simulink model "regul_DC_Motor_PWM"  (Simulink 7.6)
settings: Solver=ode15s  StartTime=0.0  StopTime=400  AbsTol=1e9
InitFcn:
  | clc, close all
  | N=400;
StopFcn:
  | load regul_vit_PWM.mat
  | 
  | plot(x(1,:),x(3,:), x(1,:),x(5,:))
  | grid
  | title('Consigne et sortie vitesse -  moteur DC  par pont en H et PWM')
  | xlabel('temps')
  | 
  | figure
  | plot(x(1,:),x(4,:))
  | grid
  | title('Signal de commande')
  | xlabel('temps')
  | 
  | figure
  | plot(x(1,:),x(2,:))
  | grid
  | axis([0 N -0.2 5.2])
  | title('Tension de commande PWM')
  | xlabel('temps')
undefined symbols (not defined in the file or in its folder): sigbuilder_block
libraries: fl_lib x19, nesl_utility x5, elec_lib x3

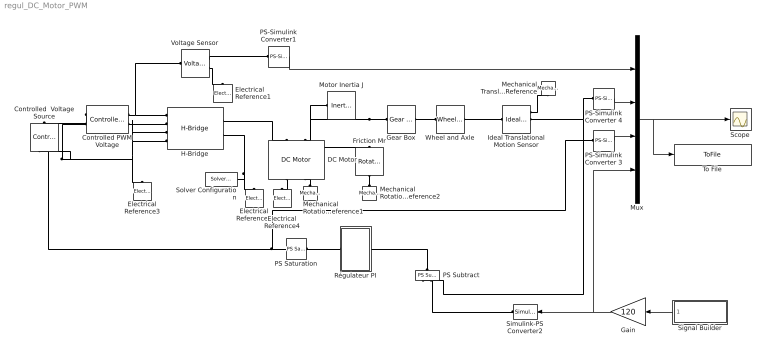
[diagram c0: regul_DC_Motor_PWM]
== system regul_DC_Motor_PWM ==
  Controlled  Voltage Source : fl_lib/Electrical/Electrical Sources/Controlled Voltage Source  DialogController=NetworkEngine.DynNeDlgSource  SystemSampleTime=-1  i_Log=off  v_Log=off  LocalVarNames=|i|v  LocalVarDescs=|i|v  LocalVarLogging=[0 0]
  Controlled PWM Voltage : elec_lib/Actuators & Drivers/Drivers/Controlled PWM Voltage  DialogController=NetworkEngine.DynNeDlgSource  SystemSampleTime=-1  F=200 Hz  Vmin=0 V  Vmax=5 V  Vm=5 V  pwm_or_av=1  current_Log=off  voltage_Log=off  power_Log=off  LocalVarNames=|current|voltage|power  LocalVarDescs=|Load current (A)|Load voltage (V)|Load power (W)  LocalVarLogging=[0 0 0]
  DC Motor : elec_lib/Actuators & Drivers/Rotational Actuators/DC Motor  DialogController=NetworkEngine.DynNeDlgSource  SystemSampleTime=-1  parameterization=1  Ra=3.9 Ohm  La=1.2e-05 H  emf_or_torque=1  Kv=7.2e-05 V/rpm  Ki=6.876e-04 N*m/A  T_stall=2.4e-04 N*m  w_max=1.91e+04 rpm  w_rated=1.5e+04 rpm  P_rated=0.08 W  V_rated=1.5 V  J=0.01 g*cm^2  lam=1e-08 N*m/(rad/s)  speed0=0 rpm  current_Log=off  voltage_Log=off  power_Log=off  i2r_Log=off  torque_Log=off  speed_Log=off  LocalVarNames=|current|voltage|power|i2r|torque|speed  LocalVarDescs=|Current (A)|Voltage (V)|Power (W)|Electrical losses (W)|Torque (Nm)|Angular speed (rad/s)  LocalVarLogging=[0 0 0 0 0 0]
  Electrical Reference{1..4} (4 alike) : fl_lib/Electrical/Electrical Elements/Electrical Reference  DialogController=NetworkEngine.DynNeDlgSource  SystemSampleTime=-1  i_Log=off  LocalVarNames=|i  LocalVarDescs=|i  LocalVarLogging=[]
  Friction Mr : fl_lib/Mechanical/Rotational Elements/Rotational Friction  DialogController=NetworkEngine.DynNeDlgSource  SystemSampleTime=-1  brkwy_trq=0.02e-3 N*m  Col_trq=0.02e-3 N*m  visc_coef=0 N*m/(rad/s)  trans_coef=10 s/rad  vel_thr=0.1 rad/s  t_Log=off  w_Log=off  LocalVarNames=|friction_torque|rel_velocity|power  LocalVarDescs=|Friction torque (N*m)|Relative velocity (rad/s)|Power (W)  LocalVarLogging=[0 0 0]
  Gain : Gain  Gain=120
  Gear Box : fl_lib/Mechanical/Mechanisms/Gear Box  DialogController=NetworkEngine.DynNeDlgSource  SystemSampleTime=-1  ratio=5  t_in_Log=off  t_out_Log=off  LocalVarNames=|t_in|t_out  LocalVarDescs=|t_in|t_out  LocalVarLogging=[0 0]
  H-Bridge : elec_lib/Actuators & Drivers/Drivers/H-Bridge  DialogController=NetworkEngine.DynNeDlgSource  SystemSampleTime=-1  Venable=2.5 V  Vmax=5 V  Vreverse=2.5 V  Vbrake=2.5 V  Vm=12 V  pwm_or_av=1  freewheeling_mode=1  Ron=0.1 Ohm  Don=0.1 Ohm  current_Log=off  voltage_Log=off  power_Log=off  LocalVarNames=|current|voltage|power  LocalVarDescs=|Load current (A)|Load voltage (V)|Load power (W)  LocalVarLogging=[0 0 0]
  Ideal Translational Motion Sensor : fl_lib/Mechanical/Mechanical Sensors/Ideal Translational Motion Sensor  DialogController=NetworkEngine.DynNeDlgSource  SystemSampleTime=-1  offset=0 m  v_Log=off  f_Log=off  x_Log=off  LocalVarNames=|v|f|x  LocalVarDescs=|v|f|x  LocalVarLogging=[0 0 0]
  Mechanical Rotational Reference1 : fl_lib/Mechanical/Rotational Elements/Mechanical Rotational Reference  DialogController=NetworkEngine.DynNeDlgSource  SystemSampleTime=-1  t_Log=off  LocalVarNames=|t  LocalVarDescs=|t  LocalVarLogging=[]
  Mechanical Rotational Reference2 : fl_lib/Mechanical/Rotational Elements/Mechanical Rotational Reference  DialogController=NetworkEngine.DynNeDlgSource  SystemSampleTime=-1  t_Log=off  LocalVarNames=|t  LocalVarDescs=|t  LocalVarLogging=[]
  Mechanical Translational Reference : fl_lib/Mechanical/Translational Elements/Mechanical Translational Reference  DialogController=NetworkEngine.DynNeDlgSource  SystemSampleTime=-1  f_Log=off  LocalVarNames=|f  LocalVarDescs=|f  LocalVarLogging=0
  Motor Inertia J : fl_lib/Mechanical/Rotational Elements/Inertia  DialogController=NetworkEngine.DynNeDlgSource  SystemSampleTime=-1  inertia=10 g*cm^2  initial_velocity=0 rad/s  t_Log=off  LocalVarNames=|torque|velocity  LocalVarDescs=|Inertia torque (N*m)|Inertia absolute velocity (rad/s)  LocalVarLogging=[0 0]
  Mux : Mux
  PS Saturation : fl_lib/Physical Signals/Nonlinear Operators/PS Saturation  DialogController=NetworkEngine.DynNeDlgSource  SystemSampleTime=-1  upper_limit=5  lower_limit=0  LocalVarLogging=[]
  PS Subtract : fl_lib/Physical Signals/Functions/PS Subtract  DialogController=NetworkEngine.DynNeDlgSource  SystemSampleTime=-1  LocalVarLogging=[]
  PS-Simulink Converter 3 : nesl_utility/PS-Simulink Converter  DialogController=NetworkEngine.DynNeUtilDlgSource  SystemSampleTime=-1  PhysicalDomain=network_engine_domain  LeftPortType=input  RightPortType=output  SubClassName=ps_output  Unit=1  AffineConversion=off
  PS-Simulink Converter 4 : nesl_utility/PS-Simulink Converter  DialogController=NetworkEngine.DynNeUtilDlgSource  SystemSampleTime=-1  PhysicalDomain=network_engine_domain  LeftPortType=input  RightPortType=output  SubClassName=ps_output  Unit=1  AffineConversion=off
  PS-Simulink Converter1 : nesl_utility/PS-Simulink Converter  DialogController=NetworkEngine.DynNeUtilDlgSource  SystemSampleTime=-1  PhysicalDomain=network_engine_domain  LeftPortType=input  RightPortType=output  SubClassName=ps_output  Unit=1  AffineConversion=off
  Régulateur PI : Subsystem
  Scope : Scope
  Signal Builder : Subsystem  Tag=STV Subsys  LoadFcn=sigbuilder_block('load');  StartFcn=sigbuilder_block('start');  StopFcn=sigbuilder_block('stop');  ClipboardFcn=sigbuilder_block('clipboard');
  Simulink-PS Converter2 : nesl_utility/Simulink-PS Converter  DialogController=NetworkEngine.DynNeUtilDlgSource  SystemSampleTime=-1  PhysicalDomain=network_engine_domain  LeftPortType=input  RightPortType=output  SubClassName=ps_input  Unit=1  AffineConversion=off  InputFilterTimeConstant=.001  UdotUserProvided=0
  Solver Configuration : nesl_utility/Solver Configuration  DialogController=NetworkEngine.DynNeUtilDlgSource  SystemSampleTime=-1  PhysicalDomain=network_engine_domain  LeftPortType=input  RightPortType=generic  SubClassName=solver  Accelerate=off  Profile=off  ResidualTolerance=1e-9  MaxNonlinIter=12  MaxModeIter=2  DoFixedCost=off  UseLocalSampling=off  DoDC=off  LinearAlgebra=Full  LocalSolverSampleTime=.001  LocalSolverChoice=NE_BACKWARD_EULER_ADVANCER  UseLocalSolver=off
  To File : ToFile  Filename=regul_vit_PWM.mat  MatrixName=x
  Voltage Sensor : fl_lib/Electrical/Electrical Sensors/Voltage Sensor  DialogController=NetworkEngine.DynNeDlgSource  SystemSampleTime=-1  i1_Log=off  v1_Log=off  LocalVarNames=|i1|v1  LocalVarDescs=|i1|v1  LocalVarLogging=[0 0]
  Wheel and Axle : fl_lib/Mechanical/Mechanisms/Wheel and Axle  DialogController=NetworkEngine.DynNeDlgSource  SystemSampleTime=-1  R=0.05 m  or=1  torque_A_Log=off  force_P_Log=off  ang_velocity_Log=off  velocity_Log=off  LocalVarNames=|torque_A|force_P|ang_velocity|velocity  LocalVarDescs=|Axle torque (N*m)|Periphery force (N)|Axle angular velocity (rad/s)|Periphery velocity (m/s)  LocalVarLogging=[0 0 0 0]
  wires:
  Mux/1 -> To File/1, Scope/1
  PS-Simulink Converter1/1 -> Mux/1
  PS-Simulink Converter 3/1 -> Mux/3
  PS-Simulink Converter 4/1 -> Mux/2
  Signal Builder/1(Signal 1) -> Gain/1
  Gain/1 -> Simulink-PS Converter2/1, Mux/4
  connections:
  Ideal Translational Motion Sensor/RConn1 -- Mechanical Translational Reference/LConn1
  Mechanical Rotational Reference1/LConn1 -- DC Motor/RConn2
  Wheel and Axle/LConn1 -- Gear Box/RConn1
  Wheel and Axle/RConn1 -- Ideal Translational Motion Sensor/LConn1
  Friction Mr/RConn1 -- Mechanical Rotational Reference2/LConn1
  DC Motor/RConn1 -- Electrical Reference4/LConn1
  H-Bridge/RConn2 -- Electrical Reference2/LConn1 -- Solver Configuration/RConn1
  Controlled PWM Voltage/RConn2 -- Controlled PWM Voltage/LConn2 -- Controlled  Voltage Source/RConn2 -- Electrical Reference3/LConn1 -- H-Bridge/LConn4 -- H-Bridge/LConn3 -- H-Bridge/LConn2
  Controlled PWM Voltage/LConn1 -- Controlled  Voltage Source/LConn1
  Voltage Sensor/RConn1 -- PS-Simulink Converter1/LConn1
  Voltage Sensor/RConn2 -- Electrical Reference1/LConn1
  H-Bridge/RConn1 -- DC Motor/LConn1
  PS-Simulink Converter 4/LConn1 -- Ideal Translational Motion Sensor/RConn2 -- PS Subtract/LConn2
  PS-Simulink Converter 3/LConn1 -- Controlled  Voltage Source/RConn1 -- PS Saturation/RConn1
  Controlled PWM Voltage/RConn1 -- H-Bridge/LConn1 -- Voltage Sensor/LConn1
  Simulink-PS Converter2/RConn1 -- PS Subtract/LConn1
  PS Subtract/RConn1 -- Régulateur PI/LConn1
  Friction Mr/LConn1 -- Gear Box/LConn1 -- DC Motor/LConn2 -- Motor Inertia J/LConn1
  PS Saturation/LConn1 -- Régulateur PI/RConn1

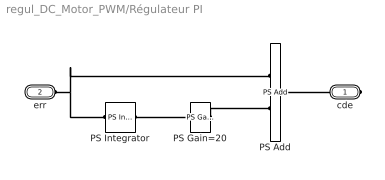
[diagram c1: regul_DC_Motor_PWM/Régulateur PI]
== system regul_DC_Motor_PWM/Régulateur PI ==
  PS Add : fl_lib/Physical Signals/Functions/PS Add  DialogController=NetworkEngine.DynNeDlgSource  SystemSampleTime=-1  LocalVarLogging=[]
  PS Gain=20 : fl_lib/Physical Signals/Functions/PS Gain  DialogController=NetworkEngine.DynNeDlgSource  SystemSampleTime=-1  gain=20  LocalVarLogging=[]
  PS Integrator : fl_lib/Physical Signals/Linear Operators/PS Integrator  DialogController=NetworkEngine.DynNeDlgSource  SystemSampleTime=-1  x0=0  x_Log=off  LocalVarNames=|x  LocalVarDescs=|x  LocalVarLogging=0
  cde : PMIOPort  Port=1  Side=Right
  err : PMIOPort  Port=2  Side=Left
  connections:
  err/RConn1 -- PS Integrator/LConn1 -- PS Add/LConn1
  PS Gain=20/RConn1 -- PS Add/LConn2
  PS Integrator/RConn1 -- PS Gain=20/LConn1
  PS Add/RConn1 -- cde/RConn1

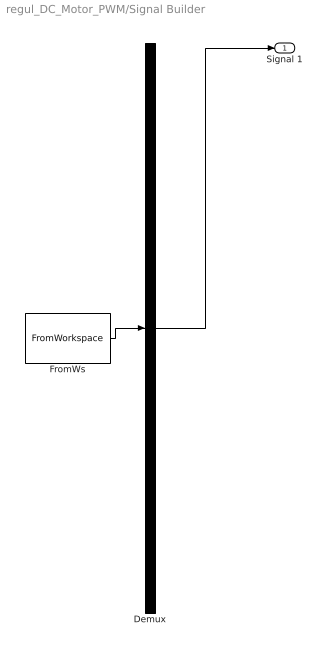
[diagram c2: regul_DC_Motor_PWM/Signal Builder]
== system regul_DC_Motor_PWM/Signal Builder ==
  Demux : Demux  Tag=STV Demux  Outputs=1
  FromWs : FromWorkspace  Tag=STV FromWs  VariableName=tuvar  SampleTime=0  SigBuilderData=DataTag0  VnvData=DataTag1
  Signal 1 : Outport  Tag=STV Outport
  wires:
  Demux/1 -> Signal 1/1
  FromWs/1 -> Demux/1
